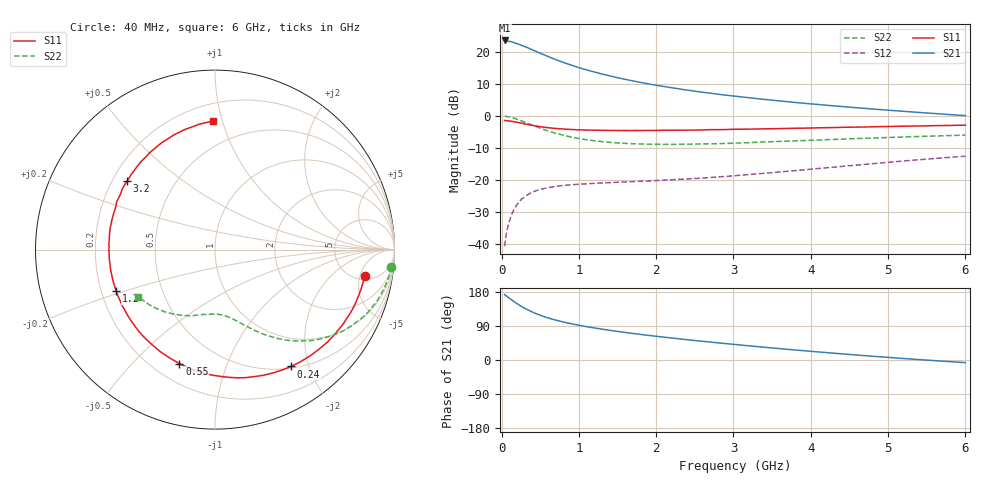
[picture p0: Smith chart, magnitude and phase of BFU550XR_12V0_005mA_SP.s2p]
! Filename:  P:\Prog\Test\Noise\ATS_data\Testdata_Net\03 Spar\BFU550XR_APG2013_45_C05_12p0V_005mA_SP_CM01_D.s2p
! Date/Time: Tue 06/Aug/2013 14:38:18
! BFU550XR_APG2013_45_C05_12p0V_1to35mA_SP_CM01_Bias4_R.s2p
! MDIF S-parameter v. bias file
! BFU550XR_APG2013_45_C05_12p0V_1to35mA_SP_CM01
! Date/time Fri Aug 02 14:58:10 2013
! VAR V_out= 12.0010
! VAR I_out= 4.9950
! VAR V_in= 0.7984
! VAR I_in= 0.0443
! Device data file deembeded for feedlines and parallel
! Original file: \03 Spar\BFU550XR_APG2013_45_C05_12p0V_005mA_SP_CM01_R.s2p
! Feed-files: PR006V01_02082013_Feed1.s2p, PR006V01_02082013_Feed2.s2p
! Parallel-file: PR006V01_02082013_Par.s2p
# MHz S MA R 50
!  Freq-MHz  S11-mag  S11-arg  S21-mag  S21-arg  S12-mag  S12-arg  S22-mag  S22-arg
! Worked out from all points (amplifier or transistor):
!   98 points, 40 MHz to 6 GHz, reference 50 ohm
!   highest |S21| = 23.6 dB at 40 MHz (marker M1)
!   |S21| within 3 dB of that: start of sweep to 406.4 MHz
!   unconditionally stable (mu >= 1): 2.446 GHz to 4.244 GHz
!   at 300 MHz: K = 0.17, MSG = 23.4 dB, |S12| = -25.2 dB
!   at 1.6 GHz: K = 0.76, MSG = 16.0 dB, |S12| = -20.6 dB
!   at 6 GHz: K = 0.84, MSG = 6.3 dB, |S12| = -12.6 dB
!   S11 on the Smith chart (normalised r, x): 40 MHz: 5.67, -5.96; 240 MHz: 0.53, -1.72; 550 MHz: 0.30, -0.69; 1.2 GHz: 0.26, -0.19; 3.2 GHz: 0.26, +0.32; 6 GHz: 0.32, +0.93
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40  0.8465 -10.1  15.06 173.0  0.009232 82.1  0.9869 -5.5
50  0.8448 -12.6  15.03 170.7  0.01145 81.6  0.9844 -7.1
140  0.818 -34.7  14.21 157.2  0.03037 70.7  0.934 -19.8
180  0.8021 -43.9  13.67 151.5  0.03773 66.1  0.9036 -24.8
240  0.7761 -57.0  12.95 143.6  0.04711 60.1  0.8525 -31.6
320  0.7405 -72.8  11.86 134.2  0.05694 53.2  0.78 -39.2
360  0.7262 -79.6  11.26 130.3  0.06098 50.4  0.747 -42.5
460  0.6905 -95.2  9.977 121.3  0.06871 44.6  0.6701 -49.3
550  0.6655 -107.3  8.991 114.4  0.07344 40.4  0.6098 -54.5
650  0.6452 -118.1  8.002 108.2  0.07764 37.2  0.559 -58.8
750  0.6299 -127.5  7.185 102.8  0.08063 34.8  0.5168 -62.5
900  0.6132 -139.4  6.216 95.7  0.0839 32.2  0.4682 -67.0
1050  0.6037 -148.9  5.449 89.8  0.08621 30.7  0.4331 -70.8
1200  0.5974 -157.1  4.845 84.6  0.0884 29.8  0.4089 -74.0
1550  0.5907 -172.5  3.832 74.1  0.0924 29.4  0.375 -80.6
2050  0.5942 171.1  2.94 61.5  0.09823 31.2  0.3593 -89.1
2500  0.5997 158.7  2.43 51.4  0.1053 33.5  0.363 -96.2
3100  0.6195 144.4  1.981 39.4  0.1187 37.1  0.3783 -105.2
3200  0.6207 142.1  1.92 37.4  0.1214 37.5  0.3818 -106.7
4100  0.6512 123.9  1.504 21.2  0.1508 39.3  0.4197 -120.4
5200  0.6901 104.0  1.178 3.9  0.1976 36.5  0.4678 -136.7
6000  0.7165 90.8  1.01 -6.9  0.2345 31.8  0.5009 -148.5
